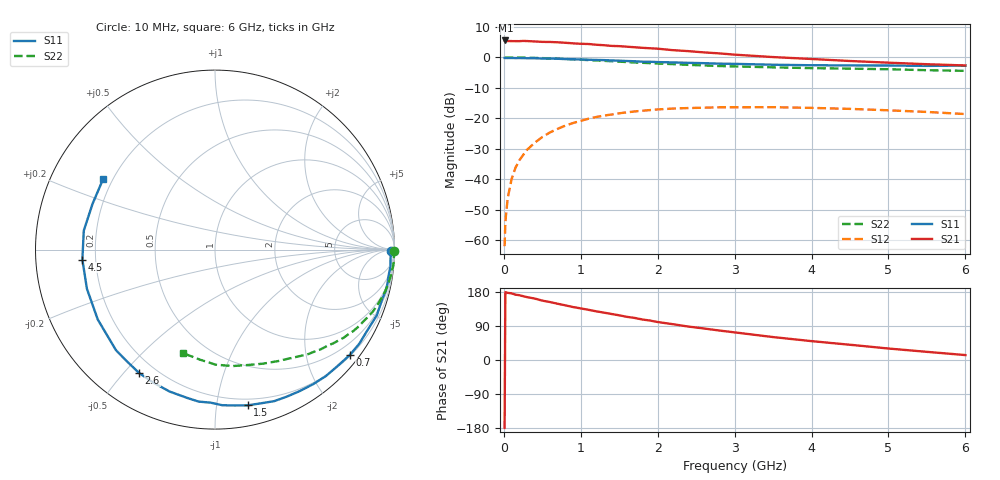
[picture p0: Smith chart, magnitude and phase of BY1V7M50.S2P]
! SIEMENS Small Signal Semiconductors
! BFY420
! Si NPN RF SIEGET Grounded Emitter Transistor in MICRO-X
! VCE = 1.75 V  IC = 0.5 mA
! Common Emitter S-Parameters:  October  1996
# GHz  S  MA  R  50
!  f  S11  S21  S12  S22
! GHz  MAG  ANG  MAG  ANG  MAG  ANG  MAG  ANG
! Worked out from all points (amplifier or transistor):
!   36 points, 10 MHz to 6 GHz, reference 50 ohm
!   highest |S21| = 5.6 dB at 20 MHz (marker M1)
!   |S21| within 3 dB of that: start of sweep to 2.122 GHz
!   unconditionally stable (mu >= 1): 4.749 GHz to end of sweep
!   at 250 MHz: K = 0.02, MSG = 18.7 dB, |S12| = -32.0 dB
!   at 1.4 GHz: K = 0.19, MSG = 11.3 dB, |S12| = -18.7 dB
!   at 6 GHz: K = 1.40, MAG = 4.2 dB, |S12| = -18.6 dB
!   S11 on the Smith chart (normalised r, x): 10 MHz: 81, -46; 700 MHz: 0.22, -2.88; 1.5 GHz: 0.15, -1.22; 2.6 GHz: 0.14, -0.55; 4.5 GHz: 0.15, -0.04; 6 GHz: 0.16, +0.28
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0.01  0.9815 -0.6  1.897 -179.2  0.0008 84.7  0.9999 -0.3
0.02  0.98 -1.3  1.904 178.9  0.002 97.5  0.9922 -0.5
0.05  0.9793 -2.9  1.861 177.2  0.0049 89.2  0.9984 -1.4
0.1  0.9819 -5.5  1.858 175.9  0.01 85.2  0.9974 -2.8
0.15  0.9784 -8.2  1.856 172.4  0.0154 84.1  0.9976 -4.2
0.2  0.9796 -11.3  1.854 171.0  0.0204 83.9  0.9963 -5.4
0.3  0.9715 -16.6  1.862 166.0  0.0304 79.3  0.9915 -8.2
0.4  0.9732 -22.1  1.832 162.2  0.0397 76.0  0.9845 -10.9
0.5  0.9612 -27.6  1.805 156.7  0.0495 72.5  0.977 -13.5
0.7  0.9533 -38.1  1.777 148.4  0.0675 66.0  0.9569 -18.6
0.9  0.9369 -48.8  1.707 139.7  0.0841 58.8  0.9328 -23.5
1.1  0.9186 -59.2  1.665 132.4  0.0989 52.5  0.9078 -28.1
1.5  0.8865 -78.2  1.535 117.9  0.1214 40.5  0.8548 -36.3
2  0.841 -100.5  1.394 100.2  0.1404 28.0  0.7965 -45.2
2.2  0.8303 -107.7  1.319 94.4  0.1452 23.2  0.7787 -48.6
2.6  0.8072 -121.6  1.213 83.2  0.15 15.4  0.7404 -54.6
3  0.7863 -134.6  1.113 72.9  0.1523 8.5  0.7137 -60.5
3.5  0.7605 -149.2  1.016 60.5  0.1529 1.2  0.6894 -67.2
4  0.7462 -163.0  0.945 49.8  0.1489 -4.9  0.6685 -74.1
4.5  0.741 -175.7  0.876 40.2  0.1434 -10.4  0.6563 -81.3
5.5  0.7284 159.5  0.776 21.5  0.1277 -17.1  0.6189 -97.8
6  0.7366 147.9  0.74 13.0  0.1179 -18.2  0.6036 -107.1
